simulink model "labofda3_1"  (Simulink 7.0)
settings: Solver=ode45  SolverMode=SingleTasking  StartTime=0.0  StopTime=30  FixedStep=0.1  RelTol=1e-3  AbsTol=1e-6
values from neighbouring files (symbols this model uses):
  D = 0.4    [labofda3.m]
  K = 1    [labofda3.m]
  M = 1    [labofda3.m]

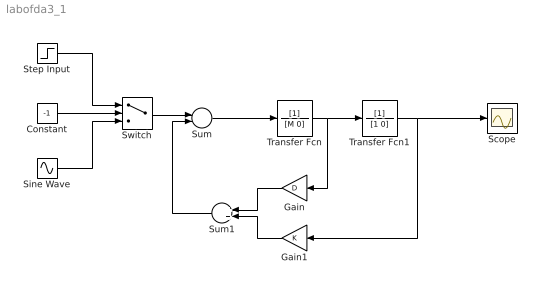
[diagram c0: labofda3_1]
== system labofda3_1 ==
  Constant : Constant  Value=-1
  Gain : Gain  Orientation=left  Gain=D
  Gain1 : Gain  Orientation=left  Gain=K
  Scope : Scope
  Sine Wave : Sin
  Step Input : Step  Time=0
  Sum : Sum  Inputs=+-
  Sum1 : Sum  Orientation=left
  Switch : Switch
  Transfer Fcn : TransferFcn  Denominator=[M 0]
  Transfer Fcn1 : TransferFcn  Denominator=[1 0]
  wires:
  Step Input/1 -> Switch/1
  Constant/1 -> Switch/2
  Sine Wave/1 -> Switch/3
  Switch/1 -> Sum/1
  Sum/1 -> Transfer Fcn/1
  Transfer Fcn/1 -> Transfer Fcn1/1, Gain/1
  Transfer Fcn1/1 -> Scope/1, Gain1/1
  Gain/1 -> Sum1/1
  Gain1/1 -> Sum1/2
  Sum1/1 -> Sum/2
